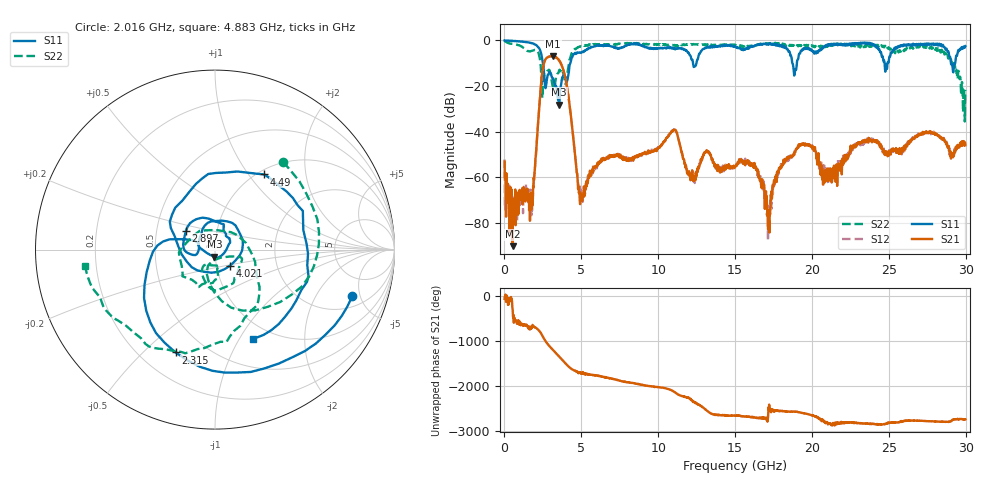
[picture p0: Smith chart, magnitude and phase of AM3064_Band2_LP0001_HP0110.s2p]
# Hz S DB R 50.0
!freq dBS11 angS11 dBS21 angS21 dBS12 angS12 dBS22 angS22
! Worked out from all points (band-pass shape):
!   1600 points, 10 MHz to 29.98 GHz, reference 50 ohm
!   highest |S21| = -6.83 dB at 3.159 GHz (marker M1); lowest = -90.2 dB at 534.8 MHz (marker M2)
!   |S21| within 3 dB of the highest: 2.574 GHz to 3.653 GHz (1.079 GHz wide, 34.7 % of centre)
!   lowest |S11| = -28.1 dB at 3.553 GHz (marker M3), VSWR 1.08, Z = 49.5 - j3.88 ohm
!   |S11| at or under -10 dB: 2.507 GHz to 4.276 GHz (1.769 GHz wide, 52.2 % of centre); 18.73 GHz to 19.02 GHz (291.8 MHz wide, 1.55 % of centre); 29.04 GHz to 29.27 GHz (225.1 MHz wide, 0.772 % of centre)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
!   |S22| runs from -35.5 to -0.2 dB; largest |S21 - S12| = 0.0099
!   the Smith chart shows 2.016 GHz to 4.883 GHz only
!   S11 on the Smith chart (normalised r, x): 2.016 GHz: 2.82, -4.24; 2.315 GHz: 0.34, -0.63; 2.897 GHz: 0.71, +0.15; 4.021 GHz: 1.17, -0.21; 4.49 GHz: 1.07, +1.19; 4.883 GHz: 0.81, -1.15
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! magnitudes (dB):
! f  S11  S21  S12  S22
! 10 MHz  0.0  -53.1  -52.2  -0.2
! 534.8 MHz  -0.2  -90.2  -69.5  -1.5
! 1.697 GHz  -1.1  -71.5  -71.6  -4.7
! 2.016 GHz  -1.8  -51.8  -53.0  -4.2
! 2.315 GHz  -4.2  -24.4  -24.3  -8.6
! 2.897 GHz  -14.3  -7.1  -7.1  -12.8
! 3.159 GHz  -16.7  -6.8  -6.9  -20.6
! 3.553 GHz  -28.1  -8.8  -8.7  -13.2
! 4.021 GHz  -18.2  -18.5  -18.4  -17.6
! 4.49 GHz  -6.0  -43.5  -43.7  -4.4
! 4.883 GHz  -5.3  -66.4  -63.8  -2.8
! 5.015 GHz  -5.3  -68.8  -66.7  -2.6
! 10 GHz  -3.4  -47.2  -47.1  -1.8
! 15 GHz  -2.6  -55.6  -55.3  -1.9
! 16.26 GHz  -2.3  -53.9  -53.7  -2.4
! 17.22 GHz  -1.3  -79.3  -80.5  -1.5
! 18 GHz  -2.7  -55.9  -54.7  -1.7
! 19.99 GHz  -4.2  -46.9  -46.8  -2.1
! 20.85 GHz  -2.7  -61.7  -60.7  -2.7
! 25 GHz  -9.1  -48.7  -48.4  -3.0
! 28.56 GHz  -2.7  -43.2  -43.2  -4.9
! 29.98 GHz  -2.5  -45.9  -45.3  -21.7
